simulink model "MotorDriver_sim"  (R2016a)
settings: Solver=FixedStepAuto  StartTime=0.0  StopTime=Endtime  FixedStep=0.05  RelTol=1e-3
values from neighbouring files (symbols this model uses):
  alpha_i = 5/37.5    (= 0.133333333333)    [MotorDriver.m]    (also in Controller.m)
  i_M_d = 3    [MotorDriver.m]    (also in MotorDriver_m.m)
  u_M_d = 10    [MotorDriver.m]
  Vs = 24    [MotorDriver.m]    (also in MotorDriver_m.m; SystemModel_noise1.m; SystemModel_noise2.m)
libraries: simulink x2

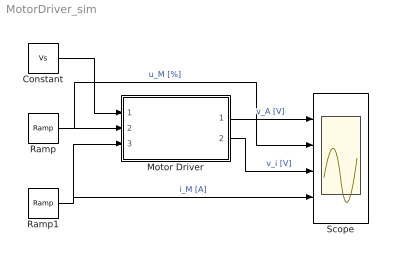
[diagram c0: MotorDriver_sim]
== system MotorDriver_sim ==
  Constant : Constant  Value=Vs
  Motor Driver : Subsystem
  Ramp : simulink/Sources/Ramp  slope=u_M_d  start=0  X0=0
  Ramp1 : simulink/Sources/Ramp  slope=i_M_d  start=0  X0=0
  Scope : Scope  NumInputPorts=4
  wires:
  Ramp/1 -> Scope/2, Motor Driver/2(u_M [%])  "u_M [%]"
  Motor Driver/1(v_A [V]) -> Scope/1  "v_A [V]"
  Constant/1 -> Motor Driver/1(Vs [V])
  Ramp1/1 -> Motor Driver/3(i_M [A]), Scope/4  "i_M [A]"
  Motor Driver/2(v_i [V]) -> Scope/3  "v_i [V]"

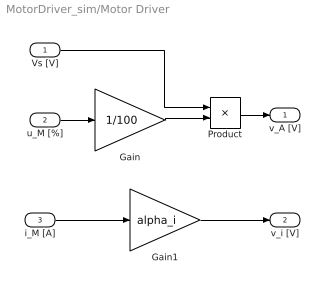
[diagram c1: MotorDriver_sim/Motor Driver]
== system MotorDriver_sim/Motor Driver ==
  Vs [V] : Inport
  u_M [%] : Inport  Port=2
  i_M [A] : Inport  Port=3
  Gain : Gain  Gain=1/100
  Gain1 : Gain  Gain=alpha_i
  Product : Product
  v_A [V] : Outport
  v_i [V] : Outport  Port=2
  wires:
  u_M [%]/1 -> Gain/1
  Product/1 -> v_A [V]/1
  Vs [V]/1 -> Product/1
  Gain/1 -> Product/2
  i_M [A]/1 -> Gain1/1
  Gain1/1 -> v_i [V]/1
